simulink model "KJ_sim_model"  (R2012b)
settings: Solver=ode45  StartTime=0.0  StopTime=86400.0  MaxStep=10  RelTol=1e-3
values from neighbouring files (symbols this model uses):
  c = 4180    [KJ_GUI.m]
  hod = 3600    [KJ_GUI.m]
  k_an = 0.5    [KJ_GUI.m]
  k_kj = 0.5    [KJ_GUI.m]
  k_sv = q_sv_pozad/q_rand    [KJ_GUI.m]
  k_tuv = 100    [KJ_GUI.m]
  k_ut = P_ut*k_ztrat*1000/deltaT    [KJ_GUI.m]
  KJ_1A = 5*hod    (= 18000)    [KJ_GUI.m]
  KJ_1B = 9*hod    (= 32400)    [KJ_GUI.m]
  KJ_2A = 16*hod    (= 57600)    [KJ_GUI.m]
  KJ_2B = 22*hod    (= 79200)    [KJ_GUI.m]
  ni1 = str2double(x)/100    [KJ_GUI.m]
  ni2 = str2double(x)/100    [KJ_GUI.m]
  P = 1/1000000    (= 1e-06)    [KJ_GUI.m]
  P_el = str2double(x)*1000    [KJ_GUI.m]
  Pel = 1/(3600*1000)    (= 2.77777777778e-07)    [KJ_GUI.m]
  Pn = str2double(x)*1000    [KJ_GUI.m]
  Pn2 = str2double(x)*1000    [KJ_GUI.m]
  q_tuv_c = 0.1    [KJ_GUI.m]
  q_ut = 0.2    [KJ_GUI.m]
  qn = 0.2    [KJ_GUI.m]
  ro = 1000    [KJ_GUI.m]
  S_ank = (2*pi*r*v/p)+(pi*r*r)    [KJ_GUI.m]
  S_anv = (2*pi*r*v/p)    [KJ_GUI.m]
  S_kj = 1    [KJ_GUI.m]
  S_tuv = 6.7/p    (= 1.11666666667)    [KJ_GUI.m]
  T0_an = 60    [KJ_GUI.m]
  T0_kj = 50    [KJ_GUI.m]
  T0_tuv = 50    [KJ_GUI.m]
  To = 20    [KJ_GUI.m]
  Tp = 22    [KJ_GUI.m]
  Tsv = 15    [KJ_GUI.m]    (also in KJgui_letni_provoz.m = evalin('base', 'Tsv'); KJgui_zimni_provoz.m = evalin('base', 'Tsv'))
  Ttuv_poz = str2double(x)    [KJ_GUI.m]
  Tut_poz = str2double(x)    [KJ_GUI.m]
  TUV_1a = str2double(x)    [KJ_GUI.m]
  TUV_1b = str2double(x)    [KJ_GUI.m]
  TUV_2a = str2double(x)    [KJ_GUI.m]
  TUV_2b = str2double(x)    [KJ_GUI.m]
  TUV_3a = str2double(x)    [KJ_GUI.m]
  TUV_3b = str2double(x)    [KJ_GUI.m]
  TUVon = str2double(TUVon_s)    [KJ_GUI.m]
  TUVsmes = str2double(TUVsmes_s)    [KJ_GUI.m]
  UT_1a = str2double(x)    [KJ_GUI.m]
  UT_1b = str2double(x)    [KJ_GUI.m]
  UT_2a = str2double(x)    [KJ_GUI.m]
  UT_2b = str2double(x)    [KJ_GUI.m]
  UT_3a = str2double(x)    [KJ_GUI.m]
  UT_3b = str2double(x)    [KJ_GUI.m]
  UTon = str2double(UTon_s)    [KJ_GUI.m]
  UTsmes = str2double(UTsmes_s)    [KJ_GUI.m]
  V = 0.708    [KJ_GUI.m]
  V_an = Vc/p    (= 0.125)    [KJ_GUI.m]
  V_kj = 0.005    [KJ_GUI.m]
  V_tuv = Vp/p    (= 0.005)    [KJ_GUI.m]
libraries: simulink x1
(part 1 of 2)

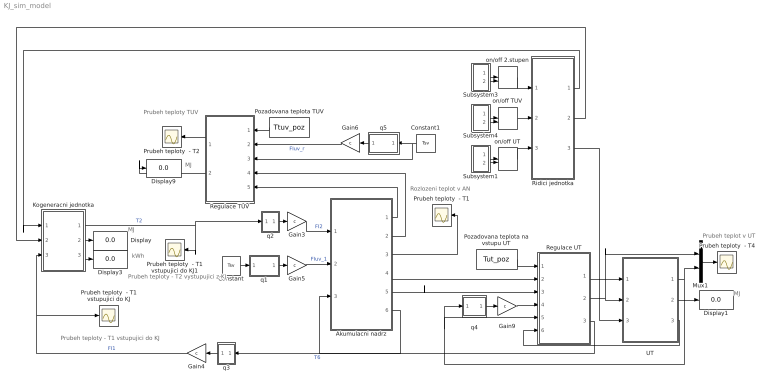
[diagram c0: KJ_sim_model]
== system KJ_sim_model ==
  note: Prubeh teplot v UT
  note: Prubeh teploty - T1 vstupujici do KJ
  note: Prubeh teploty - T2 vystupujici z KJ
  note: Rozlozeni teplot v AN
  note: kWh
  note: MJ
  note: Prubeh teploty TUV
  note: MJ
  note: MJ
  Akumulacni nadrz : Subsystem
  Constant : Constant  Value=Tsv
  Constant1 : Constant  Value=Tsv
  Display{,1,3,9} (4 alike) : Display
  Gain{3..6,9} (5 alike) : Gain  Gain=c
  Kogeneracni jednotka : Subsystem
  Mux1 : Mux  Inputs=2
  Pozadovana teplota TUV : Constant  Value=Ttuv_poz
  Pozadovana teplota na vstupu UT : Constant  Value=Tut_poz
  Prubeh teploty  - T1 : Scope
  Prubeh teploty  - T1 vstupujici do KJ : Scope
  Prubeh teploty  - T1 vstupujici do KJ1 : Scope
  Prubeh teploty  - T2 : Scope
  Prubeh teploty  - T4 : Scope
  Regulace TUV : Subsystem
  Regulace UT : Subsystem
  Ridici jednotka : Subsystem
  Subsystem1 : Subsystem
  Subsystem3 : Subsystem
  Subsystem4 : Subsystem
  UT : Subsystem
  on/off 2.stupen : ManualSwitch
  on/off TUV : ManualSwitch
  on/off UT : ManualSwitch
  q1 : Subsystem
  q2 : Subsystem
  q3 : Subsystem
  q4 : Subsystem
  q5 : Subsystem
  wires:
  Kogeneracni jednotka/1(T2) -> Prubeh teploty  - T1 vstupujici do KJ1/1, q2/1(I)  "T2"
  Kogeneracni jednotka/2(Q_kj) -> Display/1
  q2/1(" q_n ") -> Gain3/1
  Gain3/1 -> Akumulacni nadrz/1(FI2)  "FI2"
  Gain4/1 -> Prubeh teploty  - T1 vstupujici do KJ/1, Kogeneracni jednotka/3(FI1)  "FI1"
  q3/1(" q_n ") -> Gain4/1
  Akumulacni nadrz/3(Tan) -> Prubeh teploty  - T1/1
  Subsystem1/1(On) -> on/off UT/1
  Subsystem1/2(Off) -> on/off UT/2
  Subsystem3/1(On) -> on/off 2.stupen/1
  Subsystem3/2(Off) -> on/off 2.stupen/2
  Subsystem4/1(On) -> on/off TUV/1
  Subsystem4/2(Off) -> on/off TUV/2
  Kogeneracni jednotka/3(E_kj) -> Display3/1
  on/off TUV/1 -> Ridici jednotka/2(2)
  Mux1/1 -> Prubeh teploty  - T4/1
  Akumulacni nadrz/6(T6) -> q3/1(I)  "T6"
  q1/1(" q_tuv_a ") -> Gain5/1
  Constant/1 -> q1/1(I)
  Gain5/1 -> Akumulacni nadrz/2(FIuv_1)  "FIuv_1"
  Pozadovana teplota TUV/1 -> Regulace TUV/1(Ttuv_poz)
  Akumulacni nadrz/1(Tuv_2) -> Regulace TUV/5(Tuv_2)
  Gain6/1 -> Regulace TUV/2(FIuv_r)  "FIuv_r"
  Constant1/1 -> Regulace TUV/3(Tsv), q5/1(I)
  Regulace TUV/1(Tuv_3) -> Prubeh teploty  - T2/1
  on/off UT/1 -> Ridici jednotka/3(1)
  on/off 2.stupen/1 -> Ridici jednotka/1(3)
  Ridici jednotka/1("2st ") -> Kogeneracni jednotka/1(2 stupen)
  Pozadovana teplota na vstupu UT/1 -> Regulace UT/1(Tut_poz)
  q4/1(" q_ut_r") -> Gain9/1
  Gain9/1 -> Regulace UT/4(FI_ut_r)
  UT/1(Tut_2) -> Mux1/2, q4/1(I), Regulace UT/5(Tut_2)
  UT/3(FIut_2b) -> Regulace UT/6(FI_ut2b)
  Akumulacni nadrz/5(FIut_1a) -> Regulace UT/3(FIut_1a)
  Akumulacni nadrz/4(Tut_1a) -> Regulace UT/2(Tut_1a)
  Regulace UT/2(Tut_1b) -> Mux1/1, UT/2(Tut_1b)
  Regulace UT/3(Fut_2a) -> Akumulacni nadrz/3(FIut_2a)
  Regulace UT/1(FIut_1b) -> UT/1(FIut_1b)
  Ridici jednotka/2(KJ) -> Kogeneracni jednotka/2(on/off)
  Ridici jednotka/3("UT ") -> UT/3(on/off UT)
  UT/2(Q_ut) -> Display1/1
  Akumulacni nadrz/2(FIuv_2) -> Regulace TUV/4(FIuv_2)
  Regulace TUV/2(Q_tuv) -> Display9/1
  q5/1(" q_tuv_r ") -> Gain6/1

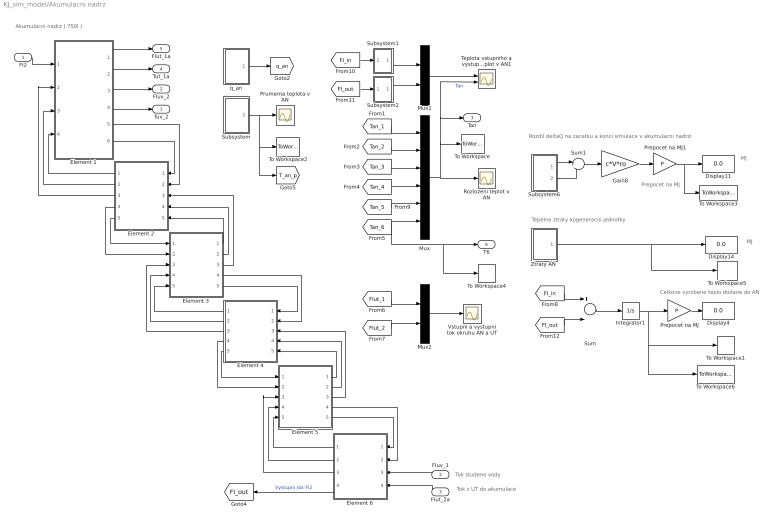
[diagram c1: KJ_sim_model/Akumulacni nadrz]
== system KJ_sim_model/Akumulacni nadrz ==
  note: Tok z UT do akumulace
  note: Akumulacni nadrz ( 750l )
  note: Celkove vyrobene teplo dodane do AN
  note: Tok studene vody
  note: MJ
  note: Prepocet na MJ
  note: Rozdil deltaQ na zacatku a konci simulace v akumulacni nadrzi
  note: Tepelne ztraty kogeneracni jednotky
  note: MJ
  FI2 : Inport
  FIuv_1 : Inport  Port=2
  FIut_2a : Inport  Port=3
  Display11 : Display
  Display14 : Display
  Display4 : Display
  Element 1 : Subsystem
  Element 2 : Subsystem
  Element 3 : Subsystem
  Element 4 : Subsystem
  Element 5 : Subsystem
  Element 6 : Subsystem
  Gain8 : Gain  Gain=c*V*ro
  Integrator1 : Integrator
  Mux : Mux  Inputs=6
  Mux1 : Mux  Inputs=2
  Mux2 : Mux  Inputs=2
  Prepocet na MJ : Gain  Gain=P
  Prepocet na MJ1 : Gain  Gain=P
  Prumerna teplota v AN : Scope
  Rozlozeni teplot v AN : Scope
  Subsystem : Subsystem
  Subsystem1 : Subsystem
  Subsystem2 : Subsystem
  Subsystem6 : Subsystem
  Sum : Sum  Inputs=+-
  Sum1 : Sum  Inputs=|+-
  Teplota vstupniho a vystupniho toku a rozlozeni teplot v AN1 : Scope  NumInputPorts=2
  To Workspace : ToWorkspace  VariableName=Tan  SampleTime=-1
  To Workspace1 : ToWorkspace  VariableName=Q_an  SampleTime=-1
  To Workspace2 : ToWorkspace  VariableName=Tan_p  SampleTime=-1
  To Workspace3 : ToWorkspace  VariableName=dQ_an  SampleTime=-1
  To Workspace4 : ToWorkspace  VariableName=T1  SampleTime=-1
  To Workspace5 : ToWorkspace  VariableName=Qz_an  SampleTime=-1
  To Workspace6 : ToWorkspace  VariableName=Q_an_suma  SampleTime=-1
  Vstupni a vystupni tok okruhu AN a UT : Scope
  "Ztraty AN " : Subsystem
  q_an : Subsystem
  Tuv_2 : Outport
  FIuv_2 : Outport  Port=2
  Tan : Outport  Port=3
  Tut_1a : Outport  Port=4
  FIut_1a : Outport  Port=5
  T6 : Outport  Port=6
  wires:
  Element 6/1(FIh_out) -> Element 5/5(FId_in)
  Element 5/4(FI_out) -> Element 6/2(FI_in)
  Element 5/5(FId_out) -> Element 6/1(FIh_in)
  FI2/1 -> Element 1/1(FI_in)
  Element 6/4(FI_out) -> [FI_out]  "Vystupni tok FI2"
  Mux/1 -> Rozlozeni teplot v AN/1, To Workspace/1, Teplota vstupniho a vystupniho toku a rozlozeni teplot v AN1/2, Tan/1  "Tan"
  [Tan_1] -> Mux/1
  [Tan_2] -> Mux/2
  [Tan_3] -> Mux/3
  [Tan_4] -> Mux/4
  [Tan_5] -> Mux/5
  [FI_out] -> Subsystem2/1(In1)
  [FI_in] -> Subsystem1/1(In1)
  Mux1/1 -> Teplota vstupniho a vystupniho toku a rozlozeni teplot v AN1/1
  q_an/1(q_an) -> [q_an]
  Subsystem/1(Tan_p) -> Prumerna teplota v AN/1, To Workspace2/1, [T_an_p]
  Element 5/1(FIh_out) -> Element 4/5(FId_in)
  Element 5/2(FIut_out) -> Element 4/4(FIut_in)
  Element 6/2(FIut_out) -> Element 5/4(FIut_in)
  Element 1/2(Tan_1) -> Tut_1a/1
  FIut_2a/1 -> Element 6/4(FIut_2)
  Element 4/5(FId_out) -> Element 5/1(FIh_in)
  Element 4/4(FI_out) -> Element 5/2(FI_in)
  Element 3/5(FId_out) -> Element 4/1(FIh_in)
  Element 4/1(FIh_out) -> Element 3/5(FId_in)
  Element 3/4(FI_out) -> Element 4/2(FI_in)
  Element 4/2(FIut_out) -> Element 3/4(FIut_in)
  Element 3/1(FIh_out) -> Element 2/5(FId_in)
  Element 2/5(FId_out) -> Element 3/1(FIh_in)
  Element 3/2(FIut_out) -> Element 2/4(FIut_in)
  Element 2/4(FI_out) -> Element 3/2(FI_in)
  Element 2/1(FIh_out) -> Element 1/4(FId_in)
  Element 1/6(FId_out) -> Element 2/1(FIh_in)
  Element 1/5(FI_out) -> Element 2/2(FI_in)
  Element 2/2(FIut_out) -> Element 1/3(FIut_in)
  [FIut_2] -> Mux2/2
  [FIut_1] -> Mux2/1
  Mux2/1 -> Vstupni a vystupni tok okruhu AN a UT/1
  Element 1/1(FIut_1) -> FIut_1a/1
  Subsystem2/1(T_out) -> Mux1/2
  Subsystem1/1("T_in ") -> Mux1/1
  Prepocet na MJ/1 -> Display4/1
  Integrator1/1 -> Prepocet na MJ/1, To Workspace1/1, To Workspace6/1
  [FI_in] -> Sum/1
  [FI_out] -> Sum/2
  Sum/1 -> Integrator1/1
  Element 2/3("FIuv_out ") -> Element 1/2(FIuv_in)
  Element 6/3("FIuv_out ") -> Element 5/3(FIuv_in)
  Element 5/3("FIuv_out ") -> Element 4/3(FIuv_in)
  Element 4/3("FIuv_out ") -> Element 3/3(FIuv_in)
  Element 3/3("FIuv_out ") -> Element 2/3(FIuv_in)
  FIuv_1/1 -> Element 6/3(FIuv_in)
  Element 1/3("FIuv_out ") -> FIuv_2/1
  Element 1/4(T_uv) -> Tuv_2/1
  Subsystem6/1(Tan_z) -> Sum1/1
  Subsystem6/2("Tan_k ") -> Sum1/2
  Sum1/1 -> Gain8/1
  Gain8/1 -> Prepocet na MJ1/1
  Prepocet na MJ1/1 -> To Workspace3/1, Display11/1
  [Tan_6] -> Mux/6, To Workspace4/1, T6/1
  "Ztraty AN "/1(Ztraty) -> To Workspace5/1, Display14/1

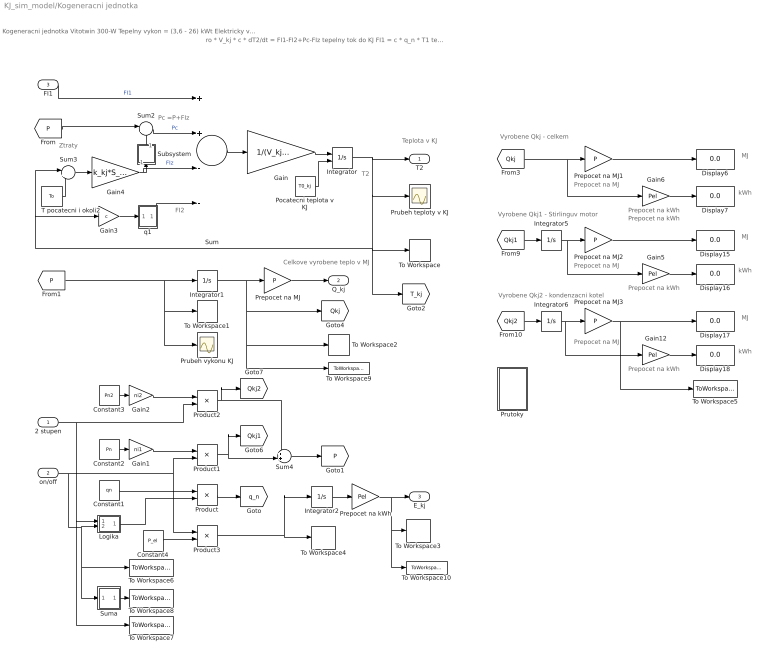
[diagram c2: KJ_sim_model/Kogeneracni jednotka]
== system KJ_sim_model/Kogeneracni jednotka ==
  note: Vyrobene Qkj1 - Stirlinguv motor
  note: Prepocet na MJ
  note: T2
  note: Teplota v KJ
  note: Ztraty
  note: Celkove vyrobene teplo v MJ
  note: ro * V_kj * c * dT2/dt = FI1-FI2+Pc-FIz tepelny tok do KJ FI1 = c * q_n * T1 tepelny tok z KJ FI2 = c * q_n * T2 celkovy vykon Pc = P + FIz Ztraty FIz = k_kj * S_kj * (T2 - To)
  note: FI2
  note: Pc =P+FIz
  note: Kogeneracni jednotka Vitotwin 300-W Tepelny vykon = (3,6 - 26) kWt Elektricky vykon = 1 kW
  note: MJ
  note: Prepocet na MJ
  note: Vyrobene Qkj2 - kondenzacni kotel
  note: kWh
  note: MJ
  note: kWh
  note: Prepocet na kWh
  note: Prepocet na kWh
  note: Prepocet na kWh
  note: Prepocet na kWh
  note: Vyrobene Qkj - celkem
  note: Prepocet na MJ
  note: MJ
  note: kWh
  2 stupen : Inport
  on/off : Inport  Port=2
  FI1 : Inport  Port=3
  Constant1 : Constant  Value=qn
  Constant2 : Constant  Value=Pn
  Constant3 : Constant  Value=Pn2
  Constant4 : Constant  Value=P_el
  Display{6..7,15..18} (6 alike) : Display
  Gain : Gain  Gain=1/(V_kj*ro*c)
  Gain1 : Gain  Gain=ni1
  Gain12 : Gain  Gain=Pel
  Gain2 : Gain  Gain=ni2
  Gain3 : Gain  Gain=c
  Gain4 : Gain  Gain=k_kj*S_kj
  Gain5 : Gain  Gain=Pel
  Gain6 : Gain  Gain=Pel
  Integrator : Integrator  InitialConditionSource=external  ZeroCross=off
  Integrator{1..2,5..6} (4 alike) : Integrator
  Logika : Subsystem
  Pocatecni teplota v KJ : Constant  Value=T0_kj
  Prepocet na MJ{,1..3} (4 alike) : Gain  Gain=P
  Prepocet na kWh : Gain  Gain=Pel
  Product{,1..3} (4 alike) : Product
  Prubeh teploty v KJ : Scope
  Prubeh vykonu KJ : Scope
  Prutoky : Subsystem
  Subsystem : Subsystem
  Sum : Sum  Inputs=++--
  Sum2 : Sum  Inputs=|++
  Sum3 : Sum  Inputs=|+-
  Sum4 : Sum  Inputs=++|
  Suma : Subsystem
  T pocatecni i okoli2 : Constant  Value=To
  To Workspace : ToWorkspace  VariableName=T2  SampleTime=-1
  To Workspace1 : ToWorkspace  VariableName=P_kj  SampleTime=-1
  To Workspace10 : ToWorkspace  VariableName=E_kj_suma  SampleTime=-1
  To Workspace2 : ToWorkspace  VariableName=Q_kj  SampleTime=-1
  To Workspace3 : ToWorkspace  VariableName=E_kj  SampleTime=-1
  To Workspace4 : ToWorkspace  VariableName=Pel_kj  SampleTime=-1
  To Workspace5 : ToWorkspace  VariableName=Q_kj2  SampleTime=-1
  To Workspace6 : ToWorkspace  VariableName=KJ_1stupen  SampleTime=-1
  To Workspace7 : ToWorkspace  VariableName=KJ_2stupen  SampleTime=-1
  To Workspace8 : ToWorkspace  VariableName=provoz_KJ  SampleTime=-1
  To Workspace9 : ToWorkspace  VariableName=Q_kj_suma  SampleTime=-1
  q1 : Subsystem
  T2 : Outport
  Q_kj : Outport  Port=2
  E_kj : Outport  Port=3
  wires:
  Integrator/1 -> T2/1, Prubeh teploty v KJ/1, Gain3/1, Sum3/1, To Workspace/1, [T_kj]
  Gain3/1 -> q1/1(I)
  Sum/1 -> Gain/1
  Gain/1 -> Integrator/1
  Pocatecni teplota v KJ/1 -> Integrator/2
  FI1/1 -> Sum/1  "FI1"
  Product/1 -> [q_n]
  Constant2/1 -> Gain1/1
  T pocatecni i okoli2/1 -> Sum3/2
  Sum3/1 -> Gain4/1
  q1/1("q_n ") -> Sum/4
  Subsystem/1(Out1) -> Sum2/2
  [P] -> Sum2/1
  Gain4/1 -> Sum/3, Subsystem/1(In1)  "FIz"
  Prepocet na MJ/1 -> Q_kj/1
  Integrator1/1 -> To Workspace2/1, To Workspace9/1, [Qkj], Prepocet na MJ/1
  Constant3/1 -> Gain2/1
  2 stupen/1 -> Product2/2, Logika/1(In1), To Workspace7/1
  Product2/1 -> [Qkj2], Sum4/1
  Product1/1 -> [Qkj1], Sum4/2
  Sum4/1 -> [P]
  Constant4/1 -> Product3/2
  Product3/1 -> Integrator2/1, To Workspace4/1
  Prepocet na kWh/1 -> E_kj/1, To Workspace3/1, To Workspace10/1
  Integrator2/1 -> Prepocet na kWh/1
  Gain1/1 -> Product1/1
  Gain2/1 -> Product2/1
  Sum2/1 -> Sum/2  "Pc"
  Constant1/1 -> Product/1
  Logika/1(Out1) -> Product/2
  Gain5/1 -> Display16/1
  Gain12/1 -> Display18/1
  [Qkj1] -> Integrator5/1
  [Qkj2] -> Integrator6/1
  Integrator5/1 -> Gain5/1, Prepocet na MJ2/1
  Prepocet na MJ2/1 -> Display15/1
  Integrator6/1 -> Prepocet na MJ3/1, Gain12/1
  Prepocet na MJ3/1 -> To Workspace5/1, Display17/1
  on/off/1 -> Suma/1(In1), To Workspace6/1, Logika/2(" "), Product1/2, Product3/1
  Suma/1(Out1) -> To Workspace8/1
  [Qkj] -> Gain6/1, Prepocet na MJ1/1
  Gain6/1 -> Display7/1
  Prepocet na MJ1/1 -> Display6/1
  [P] -> To Workspace1/1, Prubeh vykonu KJ/1, Integrator1/1

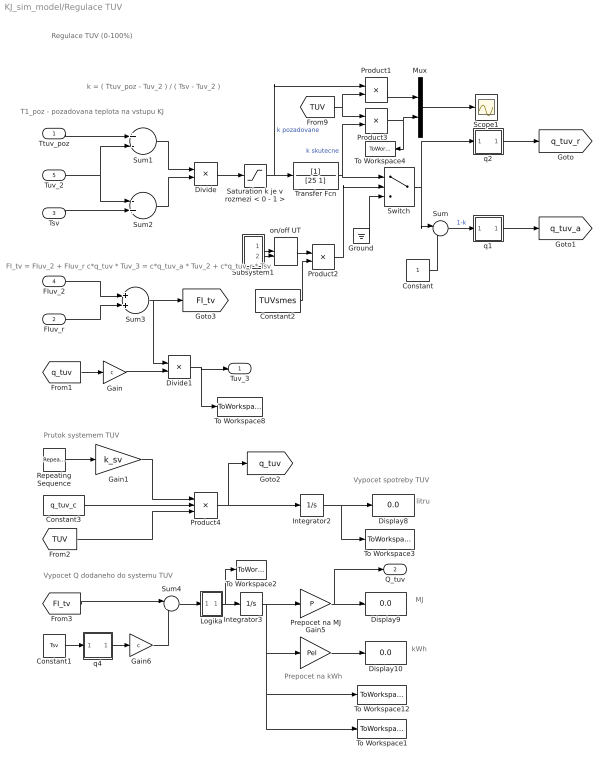
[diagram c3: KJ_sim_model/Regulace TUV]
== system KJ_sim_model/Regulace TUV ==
  note: Vypocet Q dodaneho do systemu TUV
  note: k = ( Ttuv_poz - Tuv_2 ) / ( Tsv - Tuv_2 )
  note: FI_tv = FIuv_2 + FIuv_r c*q_tuv * Tuv_3 = c*q_tuv_a * Tuv_2 + c*q_tuv_r * Tsv
  note: T1_poz - pozadovana teplota na vstupu KJ
  note: Regulace TUV (0-100%)
  note: Prepocet na kWh
  note: Vypocet spotreby TUV
  note: MJ
  note: kWh
  note: litru
  note: Prutok systemem TUV
  Ttuv_poz : Inport
  FIuv_r : Inport  Port=2
  Tsv : Inport  Port=3
  FIuv_2 : Inport  Port=4
  Tuv_2 : Inport  Port=5
  Constant : Constant
  Constant1 : Constant  Value=Tsv
  Constant2 : Constant  Value=TUVsmes
  Constant3 : Constant  Value=q_tuv_c
  Display10 : Display
  Display8 : Display
  Display9 : Display
  Divide : Product  Inputs=*/
  Divide1 : Product  Inputs=*/
  Gain : Gain  Gain=c
  Gain1 : Gain  Gain=k_sv
  Gain5 : Gain  Gain=Pel
  Gain6 : Gain  Gain=c
  Ground : Ground
  Integrator2 : Integrator
  Integrator3 : Integrator  IgnoreLimit=on
  Logika : Subsystem
  Mux : Mux  Inputs=2
  Prepocet na MJ : Gain  Gain=P
  Product1 : Product
  Product2 : Product
  Product3 : Product
  Product4 : Product  Inputs=3
  Repeating Sequence : simulink/Sources/Repeating Sequence Stair  OutValues=[0.08 0.04 0.06 0.014 0.07 0.095]  tsamp=300  OutMin=[]  OutMax=[]  OutDataTypeStr=double  OutputDataTypeScalingMode=double  OutDataType=fixdt(0,8)  ConRadixGroup=Best Precision: Vector-wise  OutScaling=2^-12
  Saturation k je v rozmezi < 0 - 1 > : Saturate  UpperLimit=1  LowerLimit=0
  Scope1 : Scope
  Subsystem1 : Subsystem
  Sum : Sum  Inputs=|-+
  Sum1 : Sum  Inputs=+-
  Sum2 : Sum  Inputs=-+
  Sum3 : Sum
  Sum4 : Sum  Inputs=|+-
  Switch : Switch  Criteria=u2 > Threshold
  To Workspace1 : ToWorkspace  VariableName=Q_tuv_suma  SampleTime=-1
  To Workspace12 : ToWorkspace  VariableName=Q_tuv  SampleTime=-1
  To Workspace2 : ToWorkspace  VariableName=P_tuv  SampleTime=-1
  To Workspace3 : ToWorkspace  VariableName=V_tuv_suma  SampleTime=-1
  To Workspace4 : ToWorkspace  VariableName=UO_tuv  SampleTime=-1
  To Workspace8 : ToWorkspace  VariableName=T_tuv  SampleTime=-1
  Transfer Fcn : TransferFcn  Denominator=[25 1]
  on/off UT : ManualSwitch
  q1 : Subsystem
  q2 : Subsystem
  q4 : Subsystem
  Tuv_3 : Outport
  Q_tuv : Outport  Port=2
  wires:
  Ttuv_poz/1 -> Sum1/1
  Tuv_2/1 -> Sum1/2, Sum2/1
  Tsv/1 -> Sum2/2
  Sum1/1 -> Divide/1
  Sum2/1 -> Divide/2
  Divide/1 -> Saturation k je v rozmezi < 0 - 1 >/1
  Transfer Fcn/1 -> Product3/2, Switch/1  "k skutecne"
  Mux/1 -> Scope1/1
  Saturation k je v rozmezi < 0 - 1 >/1 -> Transfer Fcn/1, Product1/1  "k pozadovane"
  q2/1("q_tuv ") -> [q_tuv_r]
  Constant/1 -> Sum/2
  Sum/1 -> q1/1(I)  "1-k"
  q1/1("q_tuv ") -> [q_tuv_a]
  FIuv_2/1 -> Sum3/1
  FIuv_r/1 -> Sum3/2
  Gain/1 -> Divide1/2
  Product3/1 -> To Workspace4/1, Mux/2
  Product1/1 -> Mux/1
  [TUV] -> Product3/1, Product1/2
  Subsystem1/1(On) -> on/off UT/1
  Subsystem1/2(Off) -> on/off UT/2
  Switch/1 -> Sum/1, q2/1(I)
  Ground/1 -> Switch/3
  on/off UT/1 -> Product2/1
  Constant2/1 -> Product2/2
  Product2/1 -> Switch/2
  q4/1(" q_tuv ") -> Gain6/1
  Constant1/1 -> q4/1(I)
  Divide1/1 -> To Workspace8/1, Tuv_3/1
  Integrator3/1 -> Prepocet na MJ/1, To Workspace12/1, To Workspace1/1, Gain5/1
  Prepocet na MJ/1 -> Q_tuv/1, Display9/1
  Gain5/1 -> Display10/1
  Logika/1(Out1) -> To Workspace2/1, Integrator3/1
  [q_tuv] -> Gain/1
  Integrator2/1 -> To Workspace3/1, Display8/1
  Constant3/1 -> Product4/2
  Product4/1 -> [q_tuv], Integrator2/1
  Repeating Sequence/1 -> Gain1/1
  Gain1/1 -> Product4/1
  [TUV] -> Product4/3
  Sum4/1 -> Logika/1(In1)
  Gain6/1 -> Sum4/2
  Sum3/1 -> [FI_tv], Divide1/1
  [FI_tv] -> Sum4/1

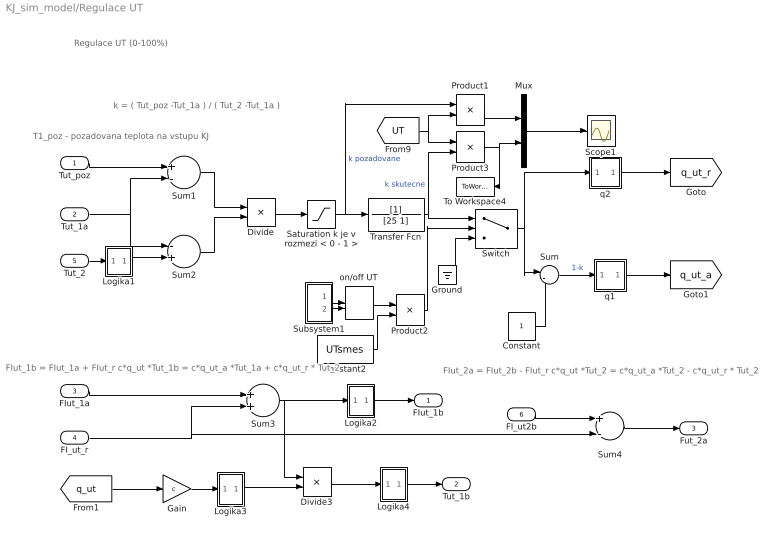
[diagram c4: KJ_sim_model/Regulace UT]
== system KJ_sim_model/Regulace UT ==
  note: k = ( Tut_poz -Tut_1a ) / ( Tut_2 -Tut_1a )
  note: FIut_1b = FIut_1a + FIut_r c*q_ut *Tut_1b = c*q_ut_a *Tut_1a + c*q_ut_r * Tut_2
  note: T1_poz - pozadovana teplota na vstupu KJ
  note: Regulace UT (0-100%)
  note: FIut_2a = FIut_2b - FIut_r c*q_ut *Tut_2 = c*q_ut_a *Tut_2 - c*q_ut_r * Tut_2
  Tut_poz : Inport
  Tut_1a : Inport  Port=2
  FIut_1a : Inport  Port=3
  FI_ut_r : Inport  Port=4
  Tut_2 : Inport  Port=5
  FI_ut2b : Inport  Port=6
  Constant : Constant
  Constant2 : Constant  Value=UTsmes
  Divide : Product  Inputs=*/
  Divide3 : Product  Inputs=*/
  Gain : Gain  Gain=c
  Ground : Ground
  Logika1 : Subsystem
  Logika2 : Subsystem
  Logika3 : Subsystem
  Logika4 : Subsystem
  Mux : Mux  Inputs=2
  Product1 : Product
  Product2 : Product
  Product3 : Product
  Saturation k je v rozmezi < 0 - 1 > : Saturate  UpperLimit=1  LowerLimit=0
  Scope1 : Scope
  Subsystem1 : Subsystem
  Sum : Sum  Inputs=|-+
  Sum1 : Sum  Inputs=+-
  Sum2 : Sum  Inputs=-+
  Sum3 : Sum
  Sum4 : Sum  Inputs=+-
  Switch : Switch  Criteria=u2 > Threshold
  To Workspace4 : ToWorkspace  VariableName=UO_ut  SampleTime=-1
  Transfer Fcn : TransferFcn  Denominator=[25 1]
  on/off UT : ManualSwitch
  q1 : Subsystem
  q2 : Subsystem
  FIut_1b : Outport
  Tut_1b : Outport  Port=2
  Fut_2a : Outport  Port=3
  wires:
  Tut_poz/1 -> Sum1/1
  Tut_1a/1 -> Sum1/2, Sum2/1
  Tut_2/1 -> Logika1/1(In1)
  Sum1/1 -> Divide/1
  Sum2/1 -> Divide/2
  Divide/1 -> Saturation k je v rozmezi < 0 - 1 >/1
  Transfer Fcn/1 -> Product3/2, Switch/1  "k skutecne"
  Mux/1 -> Scope1/1
  Saturation k je v rozmezi < 0 - 1 >/1 -> Transfer Fcn/1, Product1/1  "k pozadovane"
  q2/1("q_ut ") -> [q_ut_r]
  Constant/1 -> Sum/2
  Sum3/1 -> Divide3/1, Logika2/1(In1)
  [q_ut] -> Gain/1
  Divide3/1 -> Logika4/1(In1)
  Product3/1 -> To Workspace4/1, Mux/2
  Product1/1 -> Mux/1
  [UT] -> Product1/2, Product3/1
  Sum/1 -> q1/1(I)  "1-k"
  q1/1("q_ut ") -> [q_ut_a]
  Logika1/1(Out1) -> Sum2/2
  FI_ut2b/1 -> Sum4/1
  Sum4/1 -> Fut_2a/1
  Logika2/1(Out1) -> FIut_1b/1
  Logika4/1(Out1) -> Tut_1b/1
  FIut_1a/1 -> Sum3/1
  Gain/1 -> Logika3/1(In1)
  FI_ut_r/1 -> Sum4/2, Sum3/2
  Logika3/1(Out1) -> Divide3/2
  Subsystem1/1(On) -> on/off UT/1
  Subsystem1/2(Off) -> on/off UT/2
  Ground/1 -> Switch/3
  Product2/1 -> Switch/2
  Constant2/1 -> Product2/2
  on/off UT/1 -> Product2/1
  Switch/1 -> q2/1(I), Sum/1

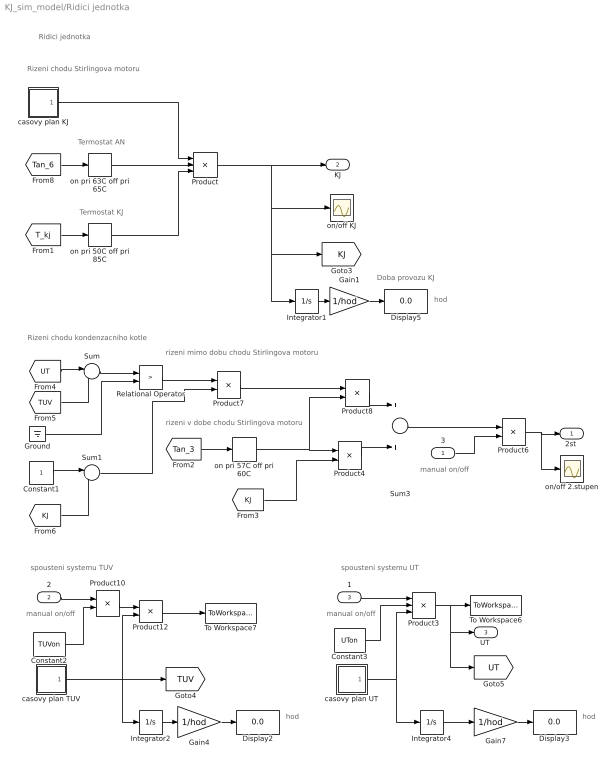
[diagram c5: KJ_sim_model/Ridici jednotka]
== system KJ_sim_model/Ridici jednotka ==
  note: hod
  note: Rizeni chodu kondenzacniho kotle
  note: Termostat AN
  note: Termostat KJ
  note: manual on/off
  note: Ridici jednotka
  note: manual on/off
  note: rizeni v dobe chodu Stirlingova motoru
  note: rizeni mimo dobu chodu Stirlingova motoru
  note: Rizeni chodu Stirlingova motoru
  note: spousteni systemu TUV
  note: manual on/off
  note: hod
  note: Doba provozu KJ
  note: hod
  note: spousteni systemu UT
  3 : Inport
  2 : Inport  Port=2
  1 : Inport  Port=3
  Constant1 : Constant
  Constant2 : Constant  Value=TUVon
  Constant3 : Constant  Value=UTon
  Display2 : Display
  Display3 : Display
  Display5 : Display
  Gain1 : Gain  Gain=1/hod
  Gain4 : Gain  Gain=1/hod
  Gain7 : Gain  Gain=1/hod
  Ground : Ground
  Integrator1 : Integrator
  Integrator2 : Integrator  IgnoreLimit=on
  Integrator4 : Integrator  IgnoreLimit=on
  Product : Product  Inputs=3
  Product{4,6..8,10,12} (6 alike) : Product
  Product3 : Product  Inputs=3
  Relational Operator : RelationalOperator  Operator=>  OutDataTypeStr=boolean
  Sum : Sum  Inputs=|++
  Sum1 : Sum  Inputs=|+-
  Sum3 : Sum
  To Workspace6 : ToWorkspace  VariableName=UT_cp  SampleTime=-1
  To Workspace7 : ToWorkspace  VariableName=TUV_cp  SampleTime=-1
  casovy plan KJ : Subsystem
  casovy plan TUV : Subsystem
  casovy plan UT : Subsystem
  on pri 50C off pri 85C : Relay  OnSwitchValue=85  OffSwitchValue=50  OnOutputValue=0  OffOutputValue=1
  on pri 57C off pri 60C : Relay  OnSwitchValue=60  OffSwitchValue=57  OnOutputValue=0  OffOutputValue=1
  on pri 63C off pri 65C : Relay  OnSwitchValue=65  OffSwitchValue=63  OnOutputValue=0  OffOutputValue=1
  on/off 2.stupen : Scope
  on/off KJ : Scope
  "2st " : Outport
  KJ : Outport  Port=2
  "UT " : Outport  Port=3
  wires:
  [Tan_6] -> on pri 63C off pri 65C/1
  [T_kj] -> on pri 50C off pri 85C/1
  on pri 50C off pri 85C/1 -> Product/3
  casovy plan KJ/1(KJ) -> Product/1
  on pri 63C off pri 65C/1 -> Product/2
  casovy plan TUV/1(TUV) -> Product12/2, [TUV], Integrator2/1
  casovy plan UT/1(UT) -> Integrator4/1, Product3/3
  Product3/1 -> [UT], "UT "/1, To Workspace6/1
  Product4/1 -> Sum3/2
  [Tan_3] -> on pri 57C off pri 60C/1
  on pri 57C off pri 60C/1 -> Product8/2, Product4/1
  Product6/1 -> on/off 2.stupen/1, "2st "/1
  3/1 -> Product6/2
  Sum3/1 -> Product6/1
  [UT] -> Sum/1
  [TUV] -> Sum/2
  Sum/1 -> Relational Operator/1
  Ground/1 -> Relational Operator/2
  Relational Operator/1 -> Product7/1
  [KJ] -> Product4/2
  Constant1/1 -> Sum1/1
  [KJ] -> Sum1/2
  Sum1/1 -> Product7/2
  Product7/1 -> Product8/1
  Product8/1 -> Sum3/1
  2/1 -> Product10/1
  Product10/1 -> Product12/1
  Constant2/1 -> Product10/2
  Constant3/1 -> Product3/2
  Gain4/1 -> Display2/1
  Integrator2/1 -> Gain4/1
  Gain7/1 -> Display3/1
  Integrator4/1 -> Gain7/1
  Product12/1 -> To Workspace7/1
  1/1 -> Product3/1
  Product/1 -> KJ/1, on/off KJ/1, Integrator1/1, [KJ]
  Integrator1/1 -> Gain1/1
  Gain1/1 -> Display5/1

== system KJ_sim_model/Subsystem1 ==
  Constant2 : Constant
  Constant3 : Constant  Value=0
  On : Outport
  Off : Outport  Port=2
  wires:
  Constant2/1 -> On/1
  Constant3/1 -> Off/1

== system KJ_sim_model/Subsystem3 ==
  Constant2 : Constant
  Constant3 : Constant  Value=0
  On : Outport
  Off : Outport  Port=2
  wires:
  Constant2/1 -> On/1
  Constant3/1 -> Off/1

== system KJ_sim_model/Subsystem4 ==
  Constant2 : Constant
  Constant3 : Constant  Value=0
  On : Outport
  Off : Outport  Port=2
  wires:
  Constant2/1 -> On/1
  Constant3/1 -> Off/1

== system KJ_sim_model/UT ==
  note: Celkove dodane teplo v MJ
  note: Ustredni topeni
  note: Vstupni tok FIut_1b = c * q_ut * Tut_1b Vystupni tok FIut_2b = c * q_ut * Tut_2 Prestup tepla UT FIut_p = k_ut * (Tut_1b - Tp)
  note: Vypocet FIut_2b FIut_1b - FIut_p = FIut_2b
  FIut_1b : Inport
  Tut_1b : Inport  Port=2
  on/off UT : Inport  Port=3
  Constant1 : Constant  Value=q_ut
  Divide : Product  Inputs=*/
  Gain : Gain  Gain=k_ut
  Gain1 : Gain  Gain=c
  Integrator1 : Integrator
  Prepocet na MJ : Gain  Gain=P
  Product1 : Product
  Product2 : Product
  Product3 : Product
  Prostorova teplota : Constant  Value=Tp
  Sum : Sum  Inputs=|+-
  Sum1 : Sum  Inputs=|+-
  To Workspace1 : ToWorkspace  VariableName=P_ut  SampleTime=-1
  To Workspace10 : ToWorkspace  VariableName=T_ut2  SampleTime=-1
  To Workspace11 : ToWorkspace  VariableName=Q_ut  SampleTime=-1
  To Workspace2 : ToWorkspace  VariableName=Q_ut_suma  SampleTime=-1
  To Workspace9 : ToWorkspace  VariableName=T_ut1  SampleTime=-1
  Tut_2 : Outport
  Q_ut : Outport  Port=2
  FIut_2b : Outport  Port=3
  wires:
  FIut_1b/1 -> Sum/1  "FIut_1b"
  Sum/1 -> Divide/1, Product2/1  "FIut_2b"
  Tut_1b/1 -> To Workspace9/1, Sum1/1
  Prostorova teplota/1 -> Sum1/2
  Sum1/1 -> Gain/1
  [q_ut] -> Gain1/1
  Gain1/1 -> Divide/2
  Divide/1 -> To Workspace10/1, Tut_2/1
  Product2/1 -> FIut_2b/1
  Constant1/1 -> Product1/2
  on/off UT/1 -> Product2/2, Product3/2, Product1/1
  Product1/1 -> [q_ut]
  Integrator1/1 -> To Workspace11/1, To Workspace2/1, Prepocet na MJ/1
  Product3/1 -> Sum/2, To Workspace1/1, Integrator1/1  "FIut_p"
  Gain/1 -> Product3/1
  Prepocet na MJ/1 -> Q_ut/1

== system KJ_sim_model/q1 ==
  I : Inport
  Product : Product
  " q_tuv_a " : Outport
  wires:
  I/1 -> Product/1
  Product/1 -> " q_tuv_a "/1
  [q_tuv_a] -> Product/2

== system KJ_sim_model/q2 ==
  I : Inport
  Product : Product
  " q_n " : Outport
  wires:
  I/1 -> Product/1
  Product/1 -> " q_n "/1
  [q_n] -> Product/2

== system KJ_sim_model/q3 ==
  I : Inport
  Product : Product
  " q_n " : Outport
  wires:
  [q_n] -> Product/2
  Product/1 -> " q_n "/1
  I/1 -> Product/1

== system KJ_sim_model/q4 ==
  I : Inport
  Logika : Subsystem
  Product : Product
  " q_ut_r" : Outport
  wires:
  I/1 -> Logika/1(In1)
  Product/1 -> " q_ut_r"/1
  [q_ut_r] -> Product/2
  Logika/1(Out1) -> Product/1

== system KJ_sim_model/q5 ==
  I : Inport
  Product : Product
  " q_tuv_r " : Outport
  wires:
  I/1 -> Product/1
  Product/1 -> " q_tuv_r "/1
  [q_tuv_r] -> Product/2

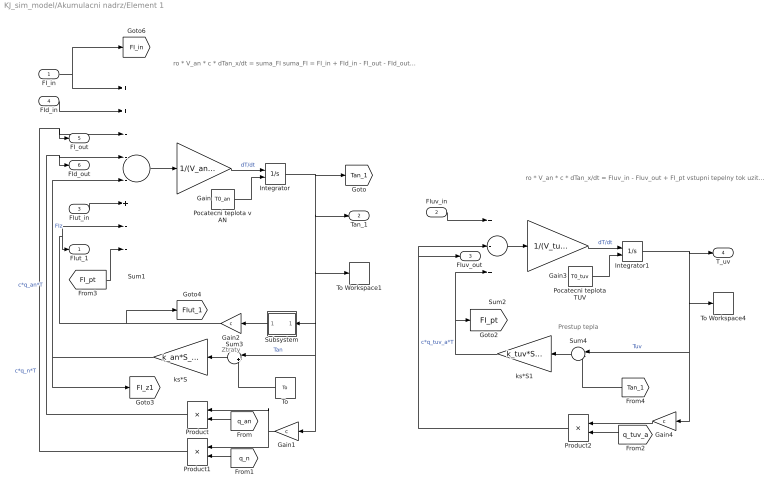
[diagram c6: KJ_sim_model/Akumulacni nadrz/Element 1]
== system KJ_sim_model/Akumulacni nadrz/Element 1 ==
  note: Ztraty
  note: Prestup tepla
  note: ro * V_an * c * dTan_x/dt = FIuv_in - FIuv_out + FI_pt vstupni tepelny tok uzitkove vody FIuv_in = c * q_tuv_a * Tuv_(x-1) vystupni tepelny tok uzitkove vody FIuv_out = c * q_tuv_a * Tuv_(x) prestup tepla z topne do uzitkove vody FI_pt = k_tuv * S_tuv * (Tan_x - Tuv_x) x ... element v akumulacni nadrzi
  note: ro * V_an * c * dTan_x/dt = suma_FI suma_FI = FI_in + FId_in - FI_out - FId_out + FIv_in - FIv_out - FIz - FI_pt tepelny tok (okruhu KJ - AN) FI_in = c * q_n * Tan_(x-1) tepelny tok (okruhu KJ - AN) FI_out = c * q_n * Tan_x vnitrni tepelny tok FId_in = c * q_an * Tan_(x+1) vnitrni tepelny tok FId_out = c * q_an * Tan_x tepelny tok (okruhu AN - UT) FIut_in = c * q_ut_a * Tan_(x+1) tepelny tok (okruhu AN - UT) FIut_out = c * q_ut_a * Tan_x tepelny tok ztrat FI_z = k_an * S_ank * (Tan_x - To) prestup tepla z topne do uzitkove vody FI_pt = k_tuv * S_tuv * (Tan_x - Tuv_x) x ... element v akumulacni nadrzi
  FI_in : Inport
  FIuv_in : Inport  Port=2
  FIut_in : Inport  Port=3
  FId_in : Inport  Port=4
  Gain : Gain  Gain=1/(V_an*ro*c)
  Gain1 : Gain  Gain=c
  Gain2 : Gain  Gain=c
  Gain3 : Gain  Gain=1/(V_tuv*ro*c)
  Gain4 : Gain  Gain=c
  Integrator : Integrator  InitialConditionSource=external  InitialCondition=30  IgnoreLimit=on
  Integrator1 : Integrator  InitialConditionSource=external  InitialCondition=30  IgnoreLimit=on
  Pocatecni teplota TUV : Constant  Value=T0_tuv
  Pocatecni teplota v AN : Constant  Value=T0_an
  Product : Product
  Product1 : Product
  Product2 : Product
  Subsystem : Subsystem
  Sum1 : Sum  Inputs=++---+--
  Sum2 : Sum  Inputs=+-+
  Sum3 : Sum  Inputs=|+-
  Sum4 : Sum  Inputs=|-+
  To : Constant  Value=To
  To Workspace1 : ToWorkspace  VariableName=Tut1a  SampleTime=-1
  To Workspace4 : ToWorkspace  VariableName=Tuv2  SampleTime=-1
  ks*S : Gain  Gain=k_an*S_ank
  ks*S1 : Gain  Gain=k_tuv*S_tuv
  FIut_1 : Outport
  Tan_1 : Outport  Port=2
  "FIuv_out " : Outport  Port=3
  T_uv : Outport  Port=4
  FI_out : Outport  Port=5
  FId_out : Outport  Port=6
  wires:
  FId_in/1 -> Sum1/2
  ks*S/1 -> [FI_z1], Sum1/5  "FIz"
  Sum3/1 -> ks*S/1
  FI_in/1 -> [FI_in], Sum1/1
  To/1 -> Sum3/2
  Gain1/1 -> Product/1, Product1/1
  Product/1 -> Sum1/4, FId_out/1  "c*q_an*T"
  Product1/1 -> Sum1/3, FI_out/1  "c*q_n*T"
  Integrator/1 -> [Tan_1], To Workspace1/1, Subsystem/1(In1), Sum3/1, Gain1/1, Tan_1/1  "Tan"
  Sum1/1 -> Gain/1
  Gain/1 -> Integrator/1  "dT/dt"
  Pocatecni teplota v AN/1 -> Integrator/2
  [q_an] -> Product/2
  [q_n] -> Product1/2
  FIut_in/1 -> Sum1/6
  Gain2/1 -> [FIut_1], FIut_1/1, Sum1/7
  [FI_pt] -> Sum1/8
  Subsystem/1(" q_ut_a") -> Gain2/1
  Gain3/1 -> Integrator1/1  "dT/dt"
  Pocatecni teplota TUV/1 -> Integrator1/2
  Sum2/1 -> Gain3/1
  FIuv_in/1 -> Sum2/1
  Product2/1 -> Sum2/2, "FIuv_out "/1  "c*q_tuv_a*T"
  Gain4/1 -> Product2/1
  [q_tuv_a] -> Product2/2
  Sum4/1 -> ks*S1/1
  Integrator1/1 -> T_uv/1, To Workspace4/1, Sum4/1, Gain4/1  "Tuv"
  ks*S1/1 -> [FI_pt], Sum2/3
  [Tan_1] -> Sum4/2

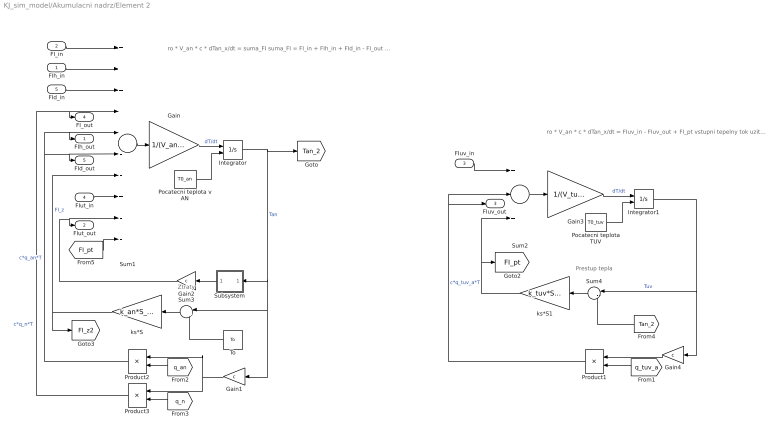
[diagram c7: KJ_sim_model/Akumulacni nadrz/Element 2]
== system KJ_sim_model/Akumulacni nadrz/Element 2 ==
  note: Ztraty
  note: ro * V_an * c * dTan_x/dt = suma_FI suma_FI = FI_in + FIh_in + FId_in - FI_out - FIh_out - FId_out + FIv_in - FIv_out - FIz - FI_pt tepelny tok (okruhu KJ - AN) FI_in = c * q_n * Tan_(x-1) tepelny tok (okruhu KJ - AN) FI_out = c * q_n * Tan_x vnitrni tepelny tok FIh_in = c * q_an * Tan_(x-1) vnitrni tepelny tok FIh_out = c * q_an * Tan_x vnitrni tepelny tok FId_in = c * q_an * Tan_(x+1) vnitrni tepelny tok FId_out = c * q_an * Tan_x tepelny tok (okruhu AN - UT) FIut_in = c * q_ut_a * Tan_(x+1) tepelny tok (okruhu AN - UT) FIut_out = c * q_ut_a * Tan_x tepelny tok ztrat FI_z = k_an * S_anv * (Tan_x - To) prestup tepla z topne do uzitkove vody FI_pt = k_tuv * S_tuv * (Tan_x - Tuv_x) x ... element v akumulacni nadrzi
  note: Prestup tepla
  note: ro * V_an * c * dTan_x/dt = FIuv_in - FIuv_out + FI_pt vstupni tepelny tok uzitkove vody FIuv_in = c * q_tuv_a * Tuv_(x-1) vystupni tepelny tok uzitkove vody FIuv_out = c * q_tuv_a * Tuv_(x) prestup tepla z topne do uzitkove vody FI_pt = k_tuv * S_tuv * (Tan_x - Tuv_x) x ... element v akumulacni nadrzi
  FIh_in : Inport
  FI_in : Inport  Port=2
  FIuv_in : Inport  Port=3
  FIut_in : Inport  Port=4
  FId_in : Inport  Port=5
  Gain : Gain  Gain=1/(V_an*ro*c)
  Gain1 : Gain  Gain=c
  Gain2 : Gain  Gain=c
  Gain3 : Gain  Gain=1/(V_tuv*ro*c)
  Gain4 : Gain  Gain=c
  Integrator : Integrator  InitialConditionSource=external  InitialCondition=30  IgnoreLimit=on
  Integrator1 : Integrator  InitialConditionSource=external  InitialCondition=30  IgnoreLimit=on
  Pocatecni teplota TUV : Constant  Value=T0_tuv
  Pocatecni teplota v AN : Constant  Value=T0_an
  Product1 : Product
  Product2 : Product
  Product3 : Product
  Subsystem : Subsystem
  Sum1 : Sum  Inputs=+++----+--
  Sum2 : Sum  Inputs=+-+
  Sum3 : Sum  Inputs=|+-
  Sum4 : Sum  Inputs=|-+
  To : Constant  Value=To
  ks*S : Gain  Gain=k_an*S_anv
  ks*S1 : Gain  Gain=k_tuv*S_tuv
  FIh_out : Outport
  FIut_out : Outport  Port=2
  "FIuv_out " : Outport  Port=3
  FI_out : Outport  Port=4
  FId_out : Outport  Port=5
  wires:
  FId_in/1 -> Sum1/3
  FIh_in/1 -> Sum1/2
  ks*S/1 -> [FI_z2], Sum1/7  "FI_z"
  Sum3/1 -> ks*S/1
  FI_in/1 -> Sum1/1
  To/1 -> Sum3/2
  Product2/1 -> FIh_out/1, Sum1/5, FId_out/1, Sum1/6  "c*q_an*T"
  Product3/1 -> FI_out/1, Sum1/4  "c*q_n*T"
  Integrator/1 -> [Tan_2], Gain1/1, Sum3/1, Subsystem/1(In1)  "Tan"
  Sum1/1 -> Gain/1
  Gain/1 -> Integrator/1  "dT/dt"
  Pocatecni teplota v AN/1 -> Integrator/2
  [q_an] -> Product2/2
  [q_n] -> Product3/2
  Gain1/1 -> Product2/1, Product3/1
  FIut_in/1 -> Sum1/8
  Gain2/1 -> FIut_out/1, Sum1/9
  Gain3/1 -> Integrator1/1  "dT/dt"
  Pocatecni teplota TUV/1 -> Integrator1/2
  Sum2/1 -> Gain3/1
  FIuv_in/1 -> Sum2/1
  Product1/1 -> Sum2/2, "FIuv_out "/1  "c*q_tuv_a*T"
  Gain4/1 -> Product1/1
  [q_tuv_a] -> Product1/2
  Sum4/1 -> ks*S1/1
  Integrator1/1 -> Sum4/1, Gain4/1  "Tuv"
  ks*S1/1 -> [FI_pt], Sum2/3
  [Tan_2] -> Sum4/2
  [FI_pt] -> Sum1/10
  Subsystem/1(" q_ut_a") -> Gain2/1

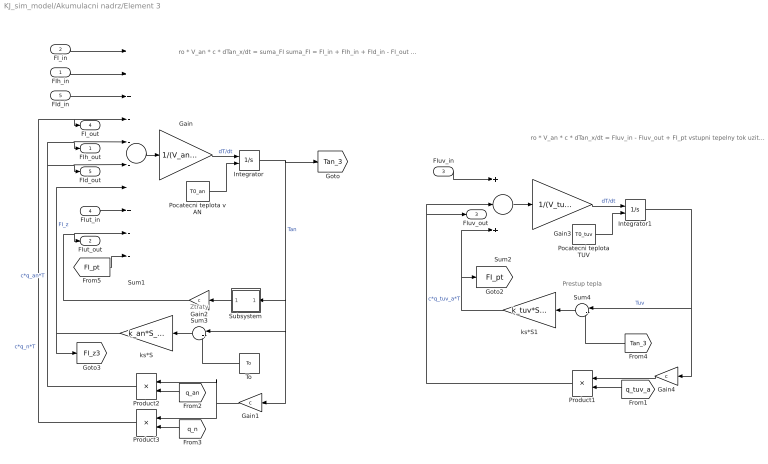
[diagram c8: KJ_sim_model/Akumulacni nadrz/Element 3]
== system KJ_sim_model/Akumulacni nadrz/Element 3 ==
  note: Ztraty
  note: ro * V_an * c * dTan_x/dt = suma_FI suma_FI = FI_in + FIh_in + FId_in - FI_out - FIh_out - FId_out + FIv_in - FIv_out - FIz - FI_pt tepelny tok (okruhu KJ - AN) FI_in = c * q_n * Tan_(x-1) tepelny tok (okruhu KJ - AN) FI_out = c * q_n * Tan_x vnitrni tepelny tok FIh_in = c * q_an * Tan_(x-1) vnitrni tepelny tok FIh_out = c * q_an * Tan_x vnitrni tepelny tok FId_in = c * q_an * Tan_(x+1) vnitrni tepelny tok FId_out = c * q_an * Tan_x tepelny tok (okruhu AN - UT) FIut_in = c * q_ut_a * Tan_(x+1) tepelny tok (okruhu AN - UT) FIut_out = c * q_ut_a * Tan_x tepelny tok ztrat FI_z = k_an * S_anv * (Tan_x - To) prestup tepla z topne do uzitkove vody FI_pt = k_tuv * S_tuv * (Tan_x - Tuv_x) x ... element v akumulacni nadrzi
  note: Prestup tepla
  note: ro * V_an * c * dTan_x/dt = FIuv_in - FIuv_out + FI_pt vstupni tepelny tok uzitkove vody FIuv_in = c * q_tuv_a * Tuv_(x-1) vystupni tepelny tok uzitkove vody FIuv_out = c * q_tuv_a * Tuv_(x) prestup tepla z topne do uzitkove vody FI_pt = k_tuv * S_tuv * (Tan_x - Tuv_x) x ... element v akumulacni nadrzi
  FIh_in : Inport
  FI_in : Inport  Port=2
  FIuv_in : Inport  Port=3
  FIut_in : Inport  Port=4
  FId_in : Inport  Port=5
  Gain : Gain  Gain=1/(V_an*ro*c)
  Gain1 : Gain  Gain=c
  Gain2 : Gain  Gain=c
  Gain3 : Gain  Gain=1/(V_tuv*ro*c)
  Gain4 : Gain  Gain=c
  Integrator : Integrator  InitialConditionSource=external  InitialCondition=30  IgnoreLimit=on
  Integrator1 : Integrator  InitialConditionSource=external  InitialCondition=30  IgnoreLimit=on
  Pocatecni teplota TUV : Constant  Value=T0_tuv
  Pocatecni teplota v AN : Constant  Value=T0_an
  Product1 : Product
  Product2 : Product
  Product3 : Product
  Subsystem : Subsystem
  Sum1 : Sum  Inputs=+++----+--
  Sum2 : Sum  Inputs=+-+
  Sum3 : Sum  Inputs=|+-
  Sum4 : Sum  Inputs=|-+
  To : Constant  Value=To
  ks*S : Gain  Gain=k_an*S_anv
  ks*S1 : Gain  Gain=k_tuv*S_tuv
  FIh_out : Outport
  FIut_out : Outport  Port=2
  "FIuv_out " : Outport  Port=3
  FI_out : Outport  Port=4
  FId_out : Outport  Port=5
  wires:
  FId_in/1 -> Sum1/3
  FIh_in/1 -> Sum1/2
  ks*S/1 -> [FI_z3], Sum1/7  "FI_z"
  Sum3/1 -> ks*S/1
  FI_in/1 -> Sum1/1
  To/1 -> Sum3/2
  Product2/1 -> FIh_out/1, Sum1/5, FId_out/1, Sum1/6  "c*q_an*T"
  Product3/1 -> FI_out/1, Sum1/4  "c*q_n*T"
  Integrator/1 -> [Tan_3], Gain1/1, Sum3/1, Subsystem/1(In1)  "Tan"
  Sum1/1 -> Gain/1
  Gain/1 -> Integrator/1  "dT/dt"
  Pocatecni teplota v AN/1 -> Integrator/2
  [q_an] -> Product2/2
  [q_n] -> Product3/2
  Gain1/1 -> Product2/1, Product3/1
  FIut_in/1 -> Sum1/8
  Gain2/1 -> FIut_out/1, Sum1/9
  Gain3/1 -> Integrator1/1  "dT/dt"
  Pocatecni teplota TUV/1 -> Integrator1/2
  Sum2/1 -> Gain3/1
  FIuv_in/1 -> Sum2/1
  Product1/1 -> Sum2/2, "FIuv_out "/1  "c*q_tuv_a*T"
  Gain4/1 -> Product1/1
  [q_tuv_a] -> Product1/2
  Sum4/1 -> ks*S1/1
  Integrator1/1 -> Sum4/1, Gain4/1  "Tuv"
  ks*S1/1 -> [FI_pt], Sum2/3
  [Tan_3] -> Sum4/2
  [FI_pt] -> Sum1/10
  Subsystem/1(" q_ut_a") -> Gain2/1

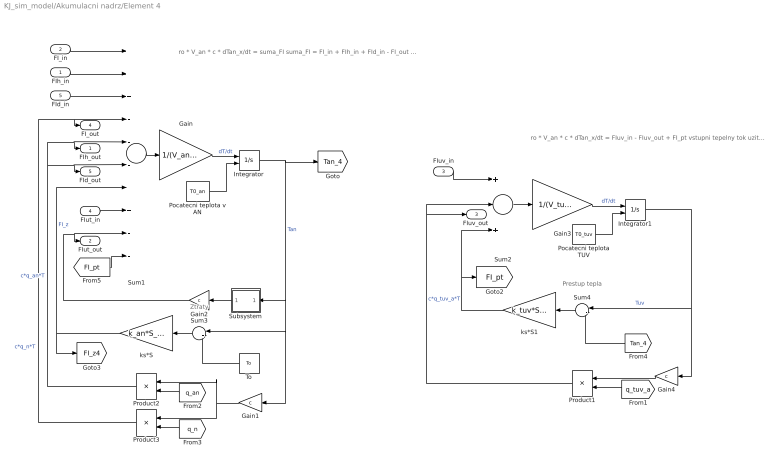
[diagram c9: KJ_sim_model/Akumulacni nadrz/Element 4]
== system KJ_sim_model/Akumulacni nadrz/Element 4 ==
  note: Ztraty
  note: ro * V_an * c * dTan_x/dt = suma_FI suma_FI = FI_in + FIh_in + FId_in - FI_out - FIh_out - FId_out + FIv_in - FIv_out - FIz - FI_pt tepelny tok (okruhu KJ - AN) FI_in = c * q_n * Tan_(x-1) tepelny tok (okruhu KJ - AN) FI_out = c * q_n * Tan_x vnitrni tepelny tok FIh_in = c * q_an * Tan_(x-1) vnitrni tepelny tok FIh_out = c * q_an * Tan_x vnitrni tepelny tok FId_in = c * q_an * Tan_(x+1) vnitrni tepelny tok FId_out = c * q_an * Tan_x tepelny tok (okruhu AN - UT) FIut_in = c * q_ut_a * Tan_(x+1) tepelny tok (okruhu AN - UT) FIut_out = c * q_ut_a * Tan_x tepelny tok ztrat FI_z = k_an * S_anv * (Tan_x - To) prestup tepla z topne do uzitkove vody FI_pt = k_tuv * S_tuv * (Tan_x - Tuv_x) x ... element v akumulacni nadrzi
  note: Prestup tepla
  note: ro * V_an * c * dTan_x/dt = FIuv_in - FIuv_out + FI_pt vstupni tepelny tok uzitkove vody FIuv_in = c * q_tuv_a * Tuv_(x-1) vystupni tepelny tok uzitkove vody FIuv_out = c * q_tuv_a * Tuv_(x) prestup tepla z topne do uzitkove vody FI_pt = k_tuv * S_tuv * (Tan_x - Tuv_x) x ... element v akumulacni nadrzi
  FIh_in : Inport
  FI_in : Inport  Port=2
  FIuv_in : Inport  Port=3
  FIut_in : Inport  Port=4
  FId_in : Inport  Port=5
  Gain : Gain  Gain=1/(V_an*ro*c)
  Gain1 : Gain  Gain=c
  Gain2 : Gain  Gain=c
  Gain3 : Gain  Gain=1/(V_tuv*ro*c)
  Gain4 : Gain  Gain=c
  Integrator : Integrator  InitialConditionSource=external  InitialCondition=30  IgnoreLimit=on
  Integrator1 : Integrator  InitialConditionSource=external  InitialCondition=30  IgnoreLimit=on
  Pocatecni teplota TUV : Constant  Value=T0_tuv
  Pocatecni teplota v AN : Constant  Value=T0_an
  Product1 : Product
  Product2 : Product
  Product3 : Product
  Subsystem : Subsystem
  Sum1 : Sum  Inputs=+++----+--
  Sum2 : Sum  Inputs=+-+
  Sum3 : Sum  Inputs=|+-
  Sum4 : Sum  Inputs=|-+
  To : Constant  Value=To
  ks*S : Gain  Gain=k_an*S_anv
  ks*S1 : Gain  Gain=k_tuv*S_tuv
  FIh_out : Outport
  FIut_out : Outport  Port=2
  "FIuv_out " : Outport  Port=3
  FI_out : Outport  Port=4
  FId_out : Outport  Port=5
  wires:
  FId_in/1 -> Sum1/3
  FIh_in/1 -> Sum1/2
  ks*S/1 -> [FI_z4], Sum1/7  "FI_z"
  Sum3/1 -> ks*S/1
  FI_in/1 -> Sum1/1
  To/1 -> Sum3/2
  Product2/1 -> FIh_out/1, Sum1/5, FId_out/1, Sum1/6  "c*q_an*T"
  Product3/1 -> FI_out/1, Sum1/4  "c*q_n*T"
  Integrator/1 -> [Tan_4], Gain1/1, Sum3/1, Subsystem/1(In1)  "Tan"
  Sum1/1 -> Gain/1
  Gain/1 -> Integrator/1  "dT/dt"
  Pocatecni teplota v AN/1 -> Integrator/2
  [q_an] -> Product2/2
  [q_n] -> Product3/2
  Gain1/1 -> Product2/1, Product3/1
  FIut_in/1 -> Sum1/8
  Gain2/1 -> FIut_out/1, Sum1/9
  Gain3/1 -> Integrator1/1  "dT/dt"
  Pocatecni teplota TUV/1 -> Integrator1/2
  Sum2/1 -> Gain3/1
  FIuv_in/1 -> Sum2/1
  Product1/1 -> Sum2/2, "FIuv_out "/1  "c*q_tuv_a*T"
  Gain4/1 -> Product1/1
  [q_tuv_a] -> Product1/2
  Sum4/1 -> ks*S1/1
  Integrator1/1 -> Sum4/1, Gain4/1  "Tuv"
  ks*S1/1 -> [FI_pt], Sum2/3
  [Tan_4] -> Sum4/2
  [FI_pt] -> Sum1/10
  Subsystem/1(" q_ut_a") -> Gain2/1

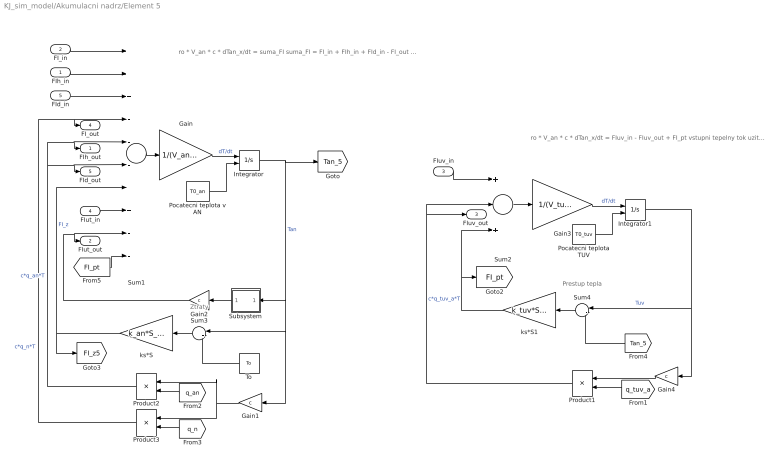
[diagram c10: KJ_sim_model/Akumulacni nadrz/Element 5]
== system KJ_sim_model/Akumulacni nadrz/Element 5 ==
  note: Ztraty
  note: ro * V_an * c * dTan_x/dt = suma_FI suma_FI = FI_in + FIh_in + FId_in - FI_out - FIh_out - FId_out + FIv_in - FIv_out - FIz - FI_pt tepelny tok (okruhu KJ - AN) FI_in = c * q_n * Tan_(x-1) tepelny tok (okruhu KJ - AN) FI_out = c * q_n * Tan_x vnitrni tepelny tok FIh_in = c * q_an * Tan_(x-1) vnitrni tepelny tok FIh_out = c * q_an * Tan_x vnitrni tepelny tok FId_in = c * q_an * Tan_(x+1) vnitrni tepelny tok FId_out = c * q_an * Tan_x tepelny tok (okruhu AN - UT) FIut_in = c * q_ut_a * Tan_(x+1) tepelny tok (okruhu AN - UT) FIut_out = c * q_ut_a * Tan_x tepelny tok ztrat FI_z = k_an * S_anv * (Tan_x - To) prestup tepla z topne do uzitkove vody FI_pt = k_tuv * S_tuv * (Tan_x - Tuv_x) x ... element v akumulacni nadrzi
  note: Prestup tepla
  note: ro * V_an * c * dTan_x/dt = FIuv_in - FIuv_out + FI_pt vstupni tepelny tok uzitkove vody FIuv_in = c * q_tuv_a * Tuv_(x-1) vystupni tepelny tok uzitkove vody FIuv_out = c * q_tuv_a * Tuv_(x) prestup tepla z topne do uzitkove vody FI_pt = k_tuv * S_tuv * (Tan_x - Tuv_x) x ... element v akumulacni nadrzi
  FIh_in : Inport
  FI_in : Inport  Port=2
  FIuv_in : Inport  Port=3
  FIut_in : Inport  Port=4
  FId_in : Inport  Port=5
  Gain : Gain  Gain=1/(V_an*ro*c)
  Gain1 : Gain  Gain=c
  Gain2 : Gain  Gain=c
  Gain3 : Gain  Gain=1/(V_tuv*ro*c)
  Gain4 : Gain  Gain=c
  Integrator : Integrator  InitialConditionSource=external  InitialCondition=30  IgnoreLimit=on
  Integrator1 : Integrator  InitialConditionSource=external  InitialCondition=30  IgnoreLimit=on
  Pocatecni teplota TUV : Constant  Value=T0_tuv
  Pocatecni teplota v AN : Constant  Value=T0_an
  Product1 : Product
  Product2 : Product
  Product3 : Product
  Subsystem : Subsystem
  Sum1 : Sum  Inputs=+++----+--
  Sum2 : Sum  Inputs=+-+
  Sum3 : Sum  Inputs=|+-
  Sum4 : Sum  Inputs=|-+
  To : Constant  Value=To
  ks*S : Gain  Gain=k_an*S_anv
  ks*S1 : Gain  Gain=k_tuv*S_tuv
  FIh_out : Outport
  FIut_out : Outport  Port=2
  "FIuv_out " : Outport  Port=3
  FI_out : Outport  Port=4
  FId_out : Outport  Port=5
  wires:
  FId_in/1 -> Sum1/3
  FIh_in/1 -> Sum1/2
  ks*S/1 -> [FI_z5], Sum1/7  "FI_z"
  Sum3/1 -> ks*S/1
  FI_in/1 -> Sum1/1
  To/1 -> Sum3/2
  Product2/1 -> FIh_out/1, Sum1/5, FId_out/1, Sum1/6  "c*q_an*T"
  Product3/1 -> FI_out/1, Sum1/4  "c*q_n*T"
  Integrator/1 -> [Tan_5], Gain1/1, Sum3/1, Subsystem/1(In1)  "Tan"
  Sum1/1 -> Gain/1
  Gain/1 -> Integrator/1  "dT/dt"
  Pocatecni teplota v AN/1 -> Integrator/2
  [q_an] -> Product2/2
  [q_n] -> Product3/2
  Gain1/1 -> Product2/1, Product3/1
  FIut_in/1 -> Sum1/8
  Gain2/1 -> FIut_out/1, Sum1/9
  Gain3/1 -> Integrator1/1  "dT/dt"
  Pocatecni teplota TUV/1 -> Integrator1/2
  Sum2/1 -> Gain3/1
  FIuv_in/1 -> Sum2/1
  Product1/1 -> Sum2/2, "FIuv_out "/1  "c*q_tuv_a*T"
  Gain4/1 -> Product1/1
  [q_tuv_a] -> Product1/2
  Sum4/1 -> ks*S1/1
  Integrator1/1 -> Sum4/1, Gain4/1  "Tuv"
  ks*S1/1 -> [FI_pt], Sum2/3
  [Tan_5] -> Sum4/2
  [FI_pt] -> Sum1/10
  Subsystem/1(" q_ut_a") -> Gain2/1

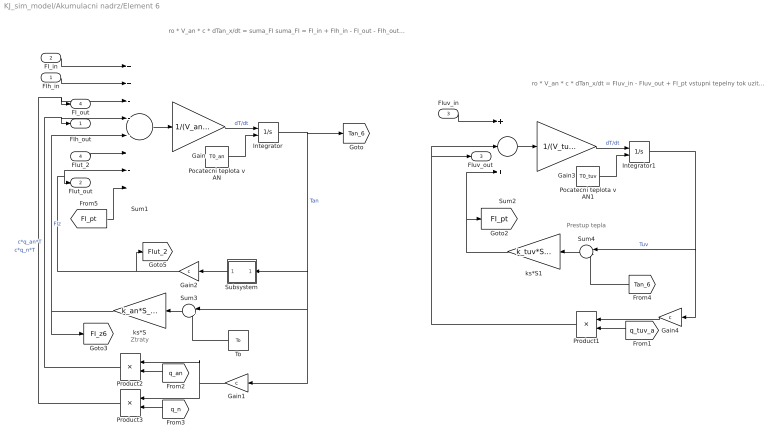
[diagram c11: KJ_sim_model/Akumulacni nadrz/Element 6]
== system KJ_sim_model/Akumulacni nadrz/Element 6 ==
  note: Ztraty
  note: Prestup tepla
  note: ro * V_an * c * dTan_x/dt = FIuv_in - FIuv_out + FI_pt vstupni tepelny tok uzitkove vody FIuv_in = c * q_tuv_a * Tuv_(x-1) vystupni tepelny tok uzitkove vody FIuv_out = c * q_tuv_a * Tuv_(x) prestup tepla z topne do uzitkove vody FI_pt = k_tuv * S_tuv * (Tan_x - Tuv_x) x ... element v akumulacni nadrzi
  note: ro * V_an * c * dTan_x/dt = suma_FI suma_FI = FI_in + FIh_in - FI_out - FIh_out + FIv_in - FIv_out - FIz - FI_pt tepelny tok (okruhu KJ - AN) FI_in = c * q_n * Tan_(x-1) tepelny tok (okruhu KJ - AN) FI_out = c * q_n * Tan_x vnitrni tepelny tok FIh_in = c * q_an * Tan_(x-1) vnitrni tepelny tok FIh_out = c * q_an * Tan_x tepelny tok (okruhu AN - UT) FIut_in = c * q_ut_a * Tan_(x+1) tepelny tok (okruhu AN - UT) FIut_out = c * q_ut_a * Tan_x tepelny tok ztrat FI_z = k_an * S_ank * (Tan_x - To) prestup tepla z topne do uzitkove vody FI_pt = k_tuv * S_tuv * (Tan_x - Tuv_x) x ... element v akumulacni nadrzi
  FIh_in : Inport
  FI_in : Inport  Port=2
  FIuv_in : Inport  Port=3
  FIut_2 : Inport  Port=4
  Gain : Gain  Gain=1/(V_an*ro*c)
  Gain1 : Gain  Gain=c
  Gain2 : Gain  Gain=c
  Gain3 : Gain  Gain=1/(V_tuv*ro*c)
  Gain4 : Gain  Gain=c
  Integrator : Integrator  InitialConditionSource=external  InitialCondition=30  IgnoreLimit=on
  Integrator1 : Integrator  InitialConditionSource=external  InitialCondition=30  IgnoreLimit=on
  Pocatecni teplota v AN : Constant  Value=T0_an
  Pocatecni teplota v AN1 : Constant  Value=T0_tuv
  Product1 : Product
  Product2 : Product
  Product3 : Product
  Subsystem : Subsystem
  Sum1 : Sum  Inputs=++---+--
  Sum2 : Sum  Inputs=+-+
  Sum3 : Sum  Inputs=|+-
  Sum4 : Sum  Inputs=|-+
  To : Constant  Value=To
  ks*S : Gain  Gain=k_an*S_ank
  ks*S1 : Gain  Gain=k_tuv*S_tuv
  FIh_out : Outport
  FIut_out : Outport  Port=2
  "FIuv_out " : Outport  Port=3
  FI_out : Outport  Port=4
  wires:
  Pocatecni teplota v AN/1 -> Integrator/2
  Gain/1 -> Integrator/1  "dT/dt"
  Sum1/1 -> Gain/1
  Integrator/1 -> [Tan_6], Subsystem/1(In1), Sum3/1, Gain1/1  "Tan"
  Product3/1 -> FI_out/1, Sum1/3  "c*q_n*T"
  Product2/1 -> FIh_out/1, Sum1/4  "c*q_an*T"
  To/1 -> Sum3/2
  FI_in/1 -> Sum1/1
  Sum3/1 -> ks*S/1
  FIh_in/1 -> Sum1/2
  [q_an] -> Product2/2
  [q_n] -> Product3/2
  Gain1/1 -> Product3/1, Product2/1
  Subsystem/1(" q_ut_a") -> Gain2/1
  ks*S/1 -> Sum1/5, [FI_z6]  "FIz"
  FIut_2/1 -> Sum1/6
  Gain2/1 -> [FIut_2], FIut_out/1, Sum1/7
  Gain3/1 -> Integrator1/1  "dT/dt"
  Pocatecni teplota v AN1/1 -> Integrator1/2
  Sum2/1 -> Gain3/1
  FIuv_in/1 -> Sum2/1
  Product1/1 -> Sum2/2, "FIuv_out "/1
  Gain4/1 -> Product1/1
  [q_tuv_a] -> Product1/2
  Sum4/1 -> ks*S1/1
  Integrator1/1 -> Sum4/1, Gain4/1  "Tuv"
  ks*S1/1 -> Sum2/3, [FI_pt]
  [Tan_6] -> Sum4/2
  [FI_pt] -> Sum1/8

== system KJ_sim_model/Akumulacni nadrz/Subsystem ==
  Gain1 : Gain  Gain=1/6
  Sum : Sum  Inputs=++++++
  Tan_p : Outport
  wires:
  Sum/1 -> Gain1/1
  Gain1/1 -> Tan_p/1
  [Tan_1] -> Sum/1
  [Tan_2] -> Sum/2
  [Tan_3] -> Sum/3
  [Tan_4] -> Sum/4
  [Tan_5] -> Sum/5
  [Tan_6] -> Sum/6

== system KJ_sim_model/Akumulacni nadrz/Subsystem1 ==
  In1 : Inport
  Divide : Product  Inputs=*/
  Gain : Gain  Gain=c
  "T_in " : Outport
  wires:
  [q_n] -> Gain/1
  Gain/1 -> Divide/2
  In1/1 -> Divide/1
  Divide/1 -> "T_in "/1

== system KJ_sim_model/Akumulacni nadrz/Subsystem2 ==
  In1 : Inport
  Divide : Product  Inputs=*/
  Gain : Gain  Gain=c
  T_out : Outport
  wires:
  Divide/1 -> T_out/1
  In1/1 -> Divide/1
  Gain/1 -> Divide/2
  [q_n] -> Gain/1

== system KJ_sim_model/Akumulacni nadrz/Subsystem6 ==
  note: T v An na zacatku simulace
  note: T v An na konci simulace
  Clock : Clock
  Display11 : Display
  Display12 : Display
  Ground : Ground
  Ground1 : Ground
  Integrator4 : Integrator  IgnoreLimit=on
  Integrator5 : Integrator  IgnoreLimit=on
  Prubeh teploty  - T6 : Scope
  Prubeh teploty  - T7 : Scope
  Switch : Switch  Criteria=u2 > Threshold  Threshold=1
  Switch1 : Switch  Criteria=u2 > Threshold  Threshold=86399
  Tan_z : Outport
  "Tan_k " : Outport  Port=2
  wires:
  [T_an_p] -> Switch/3
  Integrator4/1 -> Tan_z/1, Display12/1, Prubeh teploty  - T7/1
  Switch/1 -> Integrator4/1
  Ground/1 -> Switch/1
  Integrator5/1 -> "Tan_k "/1, Display11/1, Prubeh teploty  - T6/1
  Ground1/1 -> Switch1/3
  Clock/1 -> Switch1/2, Switch/2
  Switch1/1 -> Integrator5/1
  [T_an_p] -> Switch1/1

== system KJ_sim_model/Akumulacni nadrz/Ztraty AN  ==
  Integrator4 : Integrator  IgnoreLimit=on
  Prepocet na MJ : Gain  Gain=P
  Sum3 : Sum  Inputs=++++++
  Ztraty : Outport
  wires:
  [FI_z5] -> Sum3/5
  [FI_z4] -> Sum3/4
  [FI_z6] -> Sum3/6
  [FI_z1] -> Sum3/1
  Sum3/1 -> Integrator4/1
  Integrator4/1 -> Prepocet na MJ/1
  [FI_z2] -> Sum3/2
  [FI_z3] -> Sum3/3
  Prepocet na MJ/1 -> Ztraty/1

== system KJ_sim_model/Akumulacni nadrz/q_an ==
  Constant2 : Constant  Value=0.2
  Constant3 : Constant  Value=0.3
  Product1 : Product
  Sum1 : Sum  Inputs=+++
  q_an : Outport
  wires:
  Constant2/1 -> Sum1/2
  Product1/1 -> Sum1/1
  Constant3/1 -> Product1/2
  [q_n] -> Product1/1
  Sum1/1 -> q_an/1  "0,2+0,3*q_s+q_ut"
  [q_ut_a] -> Sum1/3

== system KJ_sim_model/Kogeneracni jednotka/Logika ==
  note: Logicka 1 - pokud je zapnut Stirling. motor nebo kotel Logicka 0 - pokud jsou vypnuty i Stirling. motor i kotel
  In1 : Inport
  " " : Inport  Port=2
  Constant : Constant
  Relational Operator : RelationalOperator  OutDataTypeStr=boolean
  Sum1 : Sum  Inputs=|++
  Out1 : Outport
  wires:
  Sum1/1 -> Relational Operator/1
  Constant/1 -> Relational Operator/2
  " "/1 -> Sum1/2
  In1/1 -> Sum1/1
  Relational Operator/1 -> Out1/1

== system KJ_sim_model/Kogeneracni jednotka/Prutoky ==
  To Workspace10 : ToWorkspace  VariableName=q_tuv_TS  SampleTime=-1
  To Workspace11 : ToWorkspace  VariableName=q_tuv_r_TS  SampleTime=-1
  To Workspace12 : ToWorkspace  VariableName=q_tuv_a_TS  SampleTime=-1
  To Workspace13 : ToWorkspace  VariableName=q_ut_TS  SampleTime=-1
  To Workspace14 : ToWorkspace  VariableName=q_ut_r_TS  SampleTime=-1
  To Workspace15 : ToWorkspace  VariableName=q_ut_a_TS  SampleTime=-1
  To Workspace9 : ToWorkspace  VariableName=q_n_TS  SampleTime=-1
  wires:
  [q_ut_a] -> To Workspace15/1
  [q_tuv_r] -> To Workspace11/1
  [q_tuv_a] -> To Workspace12/1
  [q_n] -> To Workspace9/1
  [q_tuv] -> To Workspace10/1
  [q_ut] -> To Workspace13/1
  [q_ut_r] -> To Workspace14/1

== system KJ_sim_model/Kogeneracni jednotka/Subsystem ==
  In1 : Inport
  Ground : Ground
  Integrator1 : Integrator
  Switch : Switch  Criteria=u2 > Threshold
  To Workspace9 : ToWorkspace  VariableName=Qz_kj  SampleTime=-1
  Out1 : Outport
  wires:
  [P] -> Switch/2
  Ground/1 -> Switch/3
  Switch/1 -> Out1/1
  In1/1 -> Integrator1/1, Switch/1
  Integrator1/1 -> To Workspace9/1

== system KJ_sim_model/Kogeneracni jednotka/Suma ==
  note: Prepocet na hodiny
  In1 : Inport
  Gain10 : Gain  Gain=1/hod
  Integrator4 : Integrator  IgnoreLimit=on
  Out1 : Outport
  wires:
  Integrator4/1 -> Gain10/1
  Gain10/1 -> Out1/1
  In1/1 -> Integrator4/1

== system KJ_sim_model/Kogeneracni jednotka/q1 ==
  I : Inport
  Product : Product
  "q_n " : Outport
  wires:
  I/1 -> Product/1
  Product/1 -> "q_n "/1
  [q_n] -> Product/2

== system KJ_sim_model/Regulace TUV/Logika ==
  note: Logicka 1 - pokud je zapnuty odber TUV Logicka 0 - pokud je vypnuty odber TUV
  In1 : Inport
  Ground : Ground
  Switch : Switch  Criteria=u2 > Threshold
  Out1 : Outport
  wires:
  Switch/1 -> Out1/1
  Ground/1 -> Switch/3
  In1/1 -> Switch/1
  [q_tuv] -> Switch/2

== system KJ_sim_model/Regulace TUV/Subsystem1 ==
  Constant2 : Constant
  Constant3 : Constant  Value=0
  On : Outport
  Off : Outport  Port=2
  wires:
  Constant2/1 -> On/1
  Constant3/1 -> Off/1

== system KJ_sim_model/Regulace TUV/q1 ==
  I : Inport
  Product : Product
  "q_tuv " : Outport
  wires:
  I/1 -> Product/1
  Product/1 -> "q_tuv "/1
  [q_tuv] -> Product/2
